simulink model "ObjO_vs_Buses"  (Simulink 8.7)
settings: Solver=ode1  StartTime=0.0  StopTime=10.0  RelTol=1e-3
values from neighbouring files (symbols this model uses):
  Tstep = 0.0005    [TestOrthOscObjO_init.m]    (also in TestWaveMng_init.m = 5e-05)
undefined symbols (not defined in the file or in its folder): kAB, kDiff
libraries: lib_T1Blocks_FB x1, lib_AngleBlocks x1

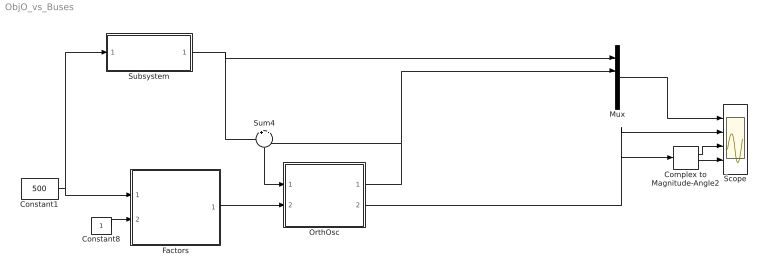
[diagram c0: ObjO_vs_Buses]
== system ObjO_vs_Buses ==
  Complex to Magnitude-Angle2 : ComplexToMagnitudeAngle
  Constant1 : Constant  Value=500  OutDataTypeStr=single
  Constant8 : Constant  OutDataTypeStr=single
  Factors : Subsystem
  Mux : Mux
  OrthOsc : Subsystem
  Scope : Scope  NumInputPorts=4
  Subsystem : Subsystem
  Sum4 : Sum  Inputs=+|-
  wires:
  Factors/1(factors) -> OrthOsc/2(In1)
  Constant8/1 -> Factors/2(In1)
  Constant1/1 -> Subsystem/1(In1), Factors/1(In4)
  Subsystem/1(Out1) -> Sum4/1, Mux/1
  Sum4/1 -> OrthOsc/1(In2)
  OrthOsc/1(Out6) -> Mux/2, Sum4/2
  OrthOsc/2(Out4) -> Complex to Magnitude-Angle2/1, Scope/2
  Mux/1 -> Scope/1
  Complex to Magnitude-Angle2/1 -> Scope/3
  Complex to Magnitude-Angle2/2 -> Scope/4

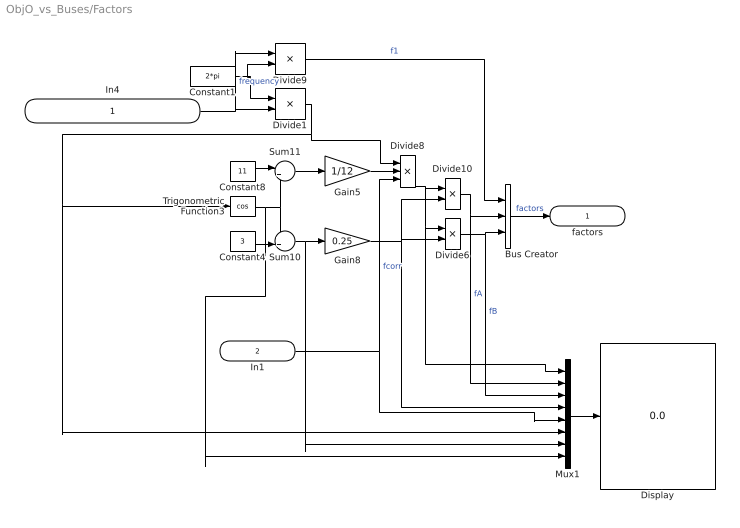
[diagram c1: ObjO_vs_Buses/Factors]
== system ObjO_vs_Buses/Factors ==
  In4 : Inport
  In1 : Inport  Port=2
  Bus Creator : BusCreator  Inputs='f1','fA','fB'
  Constant1 : Constant  Value=2*pi  OutDataTypeStr=single
  Constant4 : Constant  Value=3  OutDataTypeStr=single
  Constant8 : Constant  Value=11  OutDataTypeStr=single
  Display : Display
  Divide1 : Product  Inputs=*/
  Divide10 : Product  Inputs=*/
  Divide6 : Product  Inputs=**
  Divide8 : Product  Inputs=***
  Divide9 : Product  Inputs=*/
  Gain5 : Gain  Gain=1/12
  Gain8 : Gain  Gain=0.25
  Mux1 : Mux  Inputs=8
  Sum10 : Sum  Inputs=++|
  Sum11 : Sum  Inputs=|++
  Trigonometric Function3 : Trigonometry  Operator=cos
  factors : Outport
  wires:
  In4/1 -> Divide9/1, Divide1/2  "frequency"
  Gain5/1 -> Divide8/2
  Divide10/1 -> Bus Creator/2, Mux1/2  "fA"
  Mux1/1 -> Display/1
  Divide6/1 -> Bus Creator/3, Mux1/3  "fB"
  Divide8/1 -> Divide10/1, Mux1/1, Divide6/1
  Trigonometric Function3/1 -> Mux1/8, Sum11/2, Sum10/1
  Sum10/1 -> Mux1/7, Gain8/1
  Gain8/1 -> Mux1/4, Divide10/2, Divide6/2
  Constant8/1 -> Sum11/1
  Constant4/1 -> Sum10/2
  Sum11/1 -> Gain5/1
  In1/1 -> Divide8/3, Mux1/5  "fcorr"
  Constant1/1 -> Divide1/1, Divide9/2
  Divide1/1 -> Divide8/1, Mux1/6, Trigonometric Function3/1
  Divide9/1 -> Bus Creator/1  "f1"
  Bus Creator/1 -> factors/1  "factors"

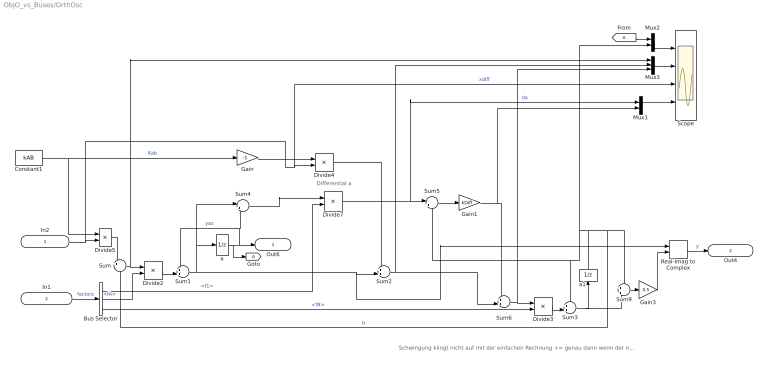
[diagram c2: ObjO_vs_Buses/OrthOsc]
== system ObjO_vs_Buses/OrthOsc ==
  note: Differential a
  note: Schwingung klingt nicht auf mit der einfachen Rechnung += genau dann wenn der neue Wert für den b-Integrator benutzt wird. Damit ist 1 Totzeit im System, neben den Integratoren. Mit 2 Totzeiten, symmetrische Schaltung, klingt die Schwingung immer auf, wenn das einfache += verwendet wird.
  In2 : Inport
  In1 : Inport  Port=2
  Bus Selector : BusSelector  OutputSignals=f1,fA,fB
  Constant1 : Constant  Value=kAB  OutDataTypeStr=single
  Divide{2..5,7} (5 alike) : Product  Inputs=**
  From : From
  Gain : Gain  Gain=-1
  Gain1 : Gain  Gain=kDiff
  Gain3 : Gain  Gain=0.5
  Goto : Goto
  Mux1 : Mux  Inputs=2
  Mux2 : Mux  Inputs=2
  Mux3 : Mux  Inputs=3
  Real-Imag to Complex : RealImagToComplex
  Scope : Scope  NumInputPorts=4
  Sum : Sum  Inputs=+|-
  Sum{1..3,6} (4 alike) : Sum  Inputs=++|
  Sum4 : Sum  Inputs=|+-
  Sum5 : Sum  Inputs=|++
  Sum9 : Sum  Inputs=+|+
  a : UnitDelay  InitialCondition=1  SampleTime=Tstep
  a1 : UnitDelay  SampleTime=Tstep
  Out6 : Outport
  Out4 : Outport  Port=2
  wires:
  In2/1 -> Scope/3, Divide4/2, Divide5/2  "xdiff"
  Sum1/1 -> Sum4/1, a/1, Real-Imag to Complex/1, Sum2/2
  Divide2/1 -> Sum1/2
  a/1 -> Out6/1, Sum4/2, Sum1/1, Goto/1  "yaz"
  Divide3/1 -> Sum3/2
  a1/1 -> Sum/2, Sum9/1, Sum5/2, Sum3/1, Mux2/2  "b"
  Sum/1 -> Mux3/1, Divide2/1
  Sum2/1 -> Sum6/2, Mux3/2
  Divide5/1 -> Sum/1
  Divide4/1 -> Sum2/1
  Bus Selector/2 -> Divide2/2  "<fA>"
  Constant1/1 -> Gain/1, Divide5/1  "Kab"
  Gain/1 -> Divide4/1
  Sum3/1 -> Sum9/2, a1/1
  Real-Imag to Complex/1 -> Out4/1  "y"
  Bus Selector/3 -> Divide3/2  "<fB>"
  Sum9/1 -> Gain3/1
  Gain3/1 -> Real-Imag to Complex/2
  Divide7/1 -> Sum5/1, Mux1/1  "da"
  Mux2/1 -> Scope/1
  Sum4/1 -> Divide7/1
  Bus Selector/1 -> Divide7/2  "<f1>"
  Mux3/1 -> Scope/2
  Sum5/1 -> Gain1/1
  Sum6/1 -> Mux3/3, Divide3/1
  In1/1 -> Bus Selector/1  "factors"
  Mux1/1 -> Scope/4
  From/1 -> Mux2/1
  Gain1/1 -> Sum6/1, Mux1/2

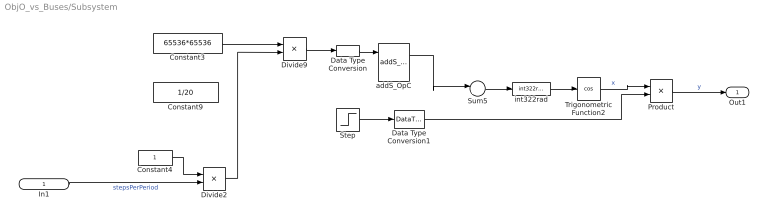
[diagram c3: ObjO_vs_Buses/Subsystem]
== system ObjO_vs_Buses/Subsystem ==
  In1 : Inport  OutDataTypeStr=single
  Constant3 : Constant  Value=65536*65536  OutDataTypeStr=single
  Constant4 : Constant  OutDataTypeStr=single
  Constant9 : Constant  Value=1/20  OutDataTypeStr=single
  Data Type Conversion : DataTypeConversion  OutDataTypeStr=int32
  Data Type Conversion1 : DataTypeConversion  OutDataTypeStr=single
  Divide2 : Product  Inputs=*/
  Divide9 : Product  Inputs=**
  Product : Product
  Step : Step  Time=1.6  Before=1  After=0.5  SampleTime=0
  Sum5 : Sum  Inputs=|++
  Trigonometric Function2 : Trigonometry  Operator=cos
  addS_OpC : lib_T1Blocks_FB/addS_OpC
  int322rad : lib_AngleBlocks/int322rad
  Out1 : Outport  OutDataTypeStr=single
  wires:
  addS_OpC/1 -> Sum5/1
  Constant3/1 -> Divide9/1
  int322rad/1 -> Trigonometric Function2/1
  Sum5/1 -> int322rad/1
  Trigonometric Function2/1 -> Product/1  "x"
  Divide9/1 -> Data Type Conversion/1
  In1/1 -> Divide2/2  "stepsPerPeriod"
  Constant4/1 -> Divide2/1
  Divide2/1 -> Divide9/2
  ? -> ?  "x"
  Data Type Conversion/1 -> addS_OpC/1
  Step/1 -> Data Type Conversion1/1
  Product/1 -> Out1/1  "y"
  Data Type Conversion1/1 -> Product/2
